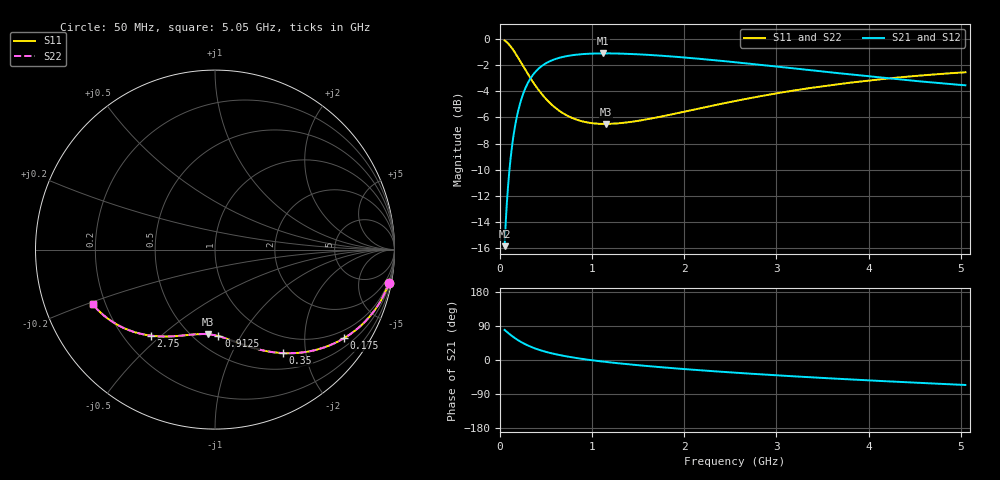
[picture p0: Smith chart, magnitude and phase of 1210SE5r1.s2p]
! AVX Thin Film Operation		Date: August 2001
! Description: Accu-P® Series, Thin Film, SMD, RF Capacitor
! Part Number: 12101J5R1ABT
! 50 MHz  -  5.05 GHz
! Serial Measurements
# mhz S db R 50
!	S11		S21		S12		S22
!	dB	Phase	dB	Phase	dB	Phase	dB	Phase
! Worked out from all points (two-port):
!   401 points, 50 MHz to 5.05 GHz, reference 50 ohm
!   highest |S21| = -1.10 dB at 1.113 GHz (marker M1); lowest = -15.8 dB at 50 MHz (marker M2)
!   |S21| within 3 dB of the highest: 256.2 MHz to end of sweep
!   lowest |S11| = -6.5 dB at 1.15 GHz (marker M3), VSWR 2.80, Z = 29.7 - j36.1 ohm
!   |S11| at or under -10 dB: nowhere
!   |S22| runs from -6.5 to -0.1 dB; largest |S21 - S12| = 0
!   S11 on the Smith chart (normalised r, x): 50 MHz: 1, -11; 175 MHz: 0.74, -3.07; 350 MHz: 0.73, -1.61; 912.5 MHz: 0.64, -0.81; 2.75 GHz: 0.31, -0.46; 5.05 GHz: 0.15, -0.21
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50  -0.12 -10.8  -15.85 79.2  -15.85 79.2  -0.12 -10.8
75  -0.25 -16.0  -12.49 74.0  -12.49 74.0  -0.25 -16.0
112.5  -0.54 -23.4  -9.30 66.6  -9.30 66.6  -0.54 -23.4
137.5  -0.78 -28.0  -7.84 62.0  -7.84 62.0  -0.78 -28.0
175  -1.18 -34.4  -6.23 55.6  -6.23 55.6  -1.18 -34.4
250  -2.07 -45.4  -4.22 44.6  -4.22 44.6  -2.07 -45.4
350  -3.21 -56.6  -2.82 33.4  -2.82 33.4  -3.21 -56.6
450  -4.19 -65.1  -2.09 24.9  -2.09 24.9  -4.19 -65.1
575  -5.11 -73.2  -1.60 16.8  -1.60 16.8  -5.11 -73.2
712.5  -5.80 -80.0  -1.33 9.9  -1.33 9.9  -5.80 -80.0
887.5  -6.29 -86.9  -1.16 3.1  -1.16 3.1  -6.29 -86.9
912.5  -6.34 -87.8  -1.15 2.2  -1.15 2.2  -6.34 -87.8
1112.5  -6.50 -94.0  -1.10 -4.0  -1.10 -4.0  -6.50 -94.0
1150  -6.50 -95.1  -1.10 -5.1  -1.10 -5.1  -6.50 -95.1
1425  -6.34 -102.0  -1.15 -12.0  -1.15 -12.0  -6.34 -102.0
1725  -5.97 -108.6  -1.27 -18.6  -1.27 -18.6  -5.97 -108.6
2125  -5.37 -116.2  -1.49 -26.2  -1.49 -26.2  -5.37 -116.2
2550  -4.75 -123.5  -1.78 -33.5  -1.78 -33.5  -4.75 -123.5
2750  -4.48 -126.6  -1.92 -36.6  -1.92 -36.6  -4.48 -126.6
3387.5  -3.73 -135.8  -2.40 -45.8  -2.40 -45.8  -3.73 -135.8
4225  -3.01 -146.5  -3.02 -56.5  -3.02 -56.5  -3.01 -146.5
5050  -2.55 -155.9  -3.54 -65.9  -3.54 -65.9  -2.55 -155.9
